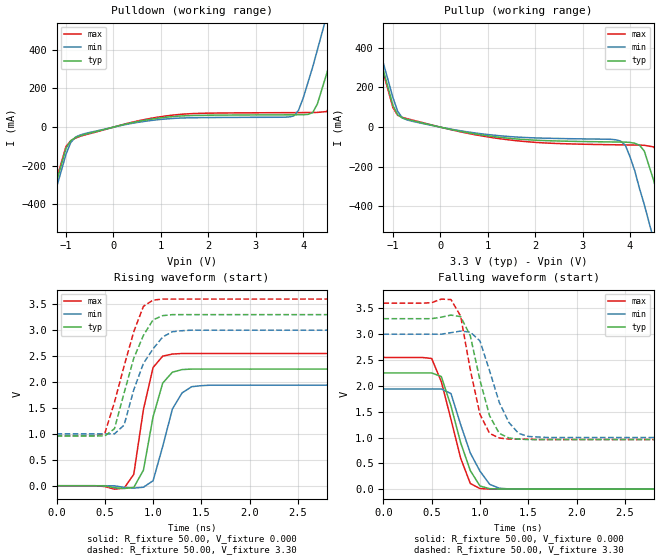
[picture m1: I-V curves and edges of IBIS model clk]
[IBIS Ver]   2.1
[File name]   66405.ibs
[File Rev]   1.0
[Date]   11/07/2011
[Source]   IDT CMD Applications Engineering
[Disclaimer] This information is for modeling purposes only, and is
(C) Copyright Integrated Circuit Systems, Inc. 1997-2004
   All rights reserved
ICS hereby grants the user of this IBIS model a non-exclusive,
nontransferable license to use this IBIS model under the following terms.
Before using this IBIS model, the user should read this license.
If the user does not accept these terms,  the IBIS model should be
returned to ICS within 30 days.
   The user is granted this license only to use the IBIS model and
is not granted rights to sell, load, rent, lease or license the IBIS
model in whole or in part, or in modified form to anyone other than
user. User may modify the IBIS model to suit its specific
applications but rights to derivative works and such modifications
shall belong to ICS.
   This IBIS model is provided on an "AS IS" basis and ICS makes
absolutely no warranty with respect to the information contained
herein. ICS DISCLAIMS AND CUSTOMER WAIVES ALL WARRANTIES, EXPRESS
OR IMPLIED, INCLUDING WARRANTIES OF MERCHANTABILITY OR FITNESS FOR
A PARTICULAR PURPOSE. The entire risk as to quality and performance
is with the Customer. ACCORDINGLY, IN NO EVENT SHALL THE COMPANY BE
LIABLE FOR ANY DAMAGES, WHETHER IN CONTRACT OR TORT,INCLUDING ANY
LOST PROFITS OR OTHER INCIDENTAL, CONSEQUENTIAL, EXEMPLARY, OR
PUNITIVE DAMAGES ARISING OUT OF THE USE OR APPLICATION OF THE IBIS
model provided in this package. Further, ICS reserves the right to
make changes without notice to any product herein to improve
reliability, function, or design. ICS does not convey any license
under patent rights or any other intellectual property rights,
including those of third parties.
   ICS is not obligated to provide maintenance or support
for the licensed IBIS model.
[Component]   ICS664-05
[Manufacturer] Integrated Circuit Systems Inc.
[Package]
|   typ   min   max
R_pkg   40m   35m   45m
L_pkg   1.65nH   1.35nH   1.95nH
C_pkg   0.24pF   0.14pF   0.34pF
[pin]   signal_name   model_name   R_pin   L_pin   C_pin
   9   CLK   clk
| Models and submodels in the file (1): clk (Output)
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|   ICS667 3.3V Clock Drive Model
| This model is suitable for all output pin on the
| ICS664-01
|   Model clk
[Model]   clk
Model_type   Output
Polarity   Non-Inverting
Vmeas =   1.65V
Cref =   5.00pF
Rref =  50.00
Vref =   1.65V
C_comp   5.50pF   5.00pF   6.00pF
[Temperature Range]   25.00   70.00   0.000
[Voltage Range]   3.30V   3.00V   3.60V
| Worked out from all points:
|   slope of the pulldown table from 0 to 0.495 V, typ, clamps not added: 17.6 ohm
|   slope of the pullup table from 0 to 0.495 V, typ, clamps not added: 20.3 ohm
|   rising waveform, R_fixture 50.00, V_fixture 0.000: 20-80 % time 158ps typ, 179ps min, 147ps max; typ from 0 V to 2.25 V
|   rising waveform, R_fixture 50.00, V_fixture 3.30: 20-80 % time 237ps typ, 252ps min, 241ps max; typ from 0.96 V to 3.3 V
|   falling waveform, R_fixture 50.00, V_fixture 0.000: 20-80 % time 217ps typ, 239ps min, 213ps max; typ from 2.25 V to 0 V
|   falling waveform, R_fixture 50.00, V_fixture 3.30: 20-80 % time 183ps typ, 225ps min, 169ps max; typ from 3.3 V to 0.96 V
[Pulldown]
| voltage   I(typ)   I(min)   I(max)
-3.3V     -2.25A     -2.28A     -2.24A
-1.5V     -540mA     -570mA     -520mA
-1V       -110mA     -140mA     -100mA
-700mV    -44.42mA   -40.49mA   -47.24mA
1.3V      55.66mA    45.68mA    63.49mA
3.8V      63.89mA    57.58mA    75.04mA
3.9V      64.06mA    85.93mA    75.17mA
4.2V      74.92mA    310mA      75.82mA
4.5V      280mA      580mA      80.87mA
4.7V      460mA      770mA      180mA
5.1V      830mA      1.14A      530mA
6.6V      2.26A      2.58A      1.96A
[Pullup]
| voltage   I(typ)   I(min)   I(max)
-3.3V     2.26A      2.29A      2.24A
-1.5V     550mA      580mA      530mA
-1V       110mA      150mA      99.39mA
-700mV    39.37mA    36.07mA    42.62mA
1.4V      -55.03mA   -46.42mA   -62.81mA
3.8V      -75.27mA   -70.05mA   -89.37mA
4V        -77.07mA   -150mA     -90.02mA
4.2V      -91.11mA   -310mA     -90.7mA
4.5V      -270mA     -570mA     -100mA
4.7V      -450mA     -760mA     -180mA
5.1V      -820mA     -1.14A     -520mA
6.6V      -2.26A     -2.57A     -1.95A
[Ramp]
| variable   typ   min   max
dV/dt_r   1.35/0.14n   1.16/0.16n   1.53/0.12n
dV/dt_f   1.40/0.18n   1.20/0.21n   1.58/0.16n
R_load = 50.00
[Rising Waveform]
R_fixture = 50.00
V_fixture = 0.000
V_fixture_min = 0.000
V_fixture_max = 0.000
| time   V(typ)   V(min)   V(max)
0s        0V         0V         0V
700ps     -53.64mV   -31.55mV   -47.01mV
800ps     -32.91mV   -45.92mV   220mV
900ps     300mV      -28.54mV   1.47V
1ns       1.33V      96.17mV    2.28V
1.1ns     1.98V      760mV      2.5V
1.2ns     2.19V      1.48V      2.54V
1.3ns     2.24V      1.79V      2.55V
1.4ns     2.25V      1.91V      2.55V
5ns       2.25V      1.94V      2.55V
[Rising Waveform]
R_fixture = 50.00
V_fixture = 3.30
V_fixture_min = 3.00
V_fixture_max = 3.60
| time   V(typ)   V(min)   V(max)
0s        960mV      1V         960mV
500ps     960mV      1V         1.01V
600ps     1.1V       1V         1.61V
700ps     1.79V      1.17V      2.31V
800ps     2.46V      1.85V      2.97V
900ps     2.9V       2.36V      3.46V
1ns       3.2V       2.64V      3.58V
1.2ns     3.3V       2.97V      3.6V
1.4ns     3.3V       3V         3.6V
5ns       3.3V       3V         3.6V
[Falling Waveform]
R_fixture = 50.00
V_fixture = 0.000
V_fixture_min = 0.000
V_fixture_max = 0.000
| time   V(typ)   V(min)   V(max)
0s        2.25V      1.94V      2.55V
500ps     2.25V      1.94V      2.53V
600ps     2.18V      1.94V      2.08V
700ps     1.61V      1.85V      1.35V
800ps     900mV      1.25V      600mV
900ps     360mV      700mV      110mV
1ns       61.1mV     350mV      11.47mV
1.1ns     9.52mV     94.71mV    2.23mV
1.3ns     1.1mV      4.55mV     810uV
5ns       3.1uV      8.72uV     1.49uV
[Falling Waveform]
R_fixture = 50.00
V_fixture = 3.30
V_fixture_min = 3.00
V_fixture_max = 3.60
| time   V(typ)   V(min)   V(max)
0s        3.3V       3V         3.6V
700ps     3.37V      3.03V      3.67V
800ps     3.34V      3.06V      3.35V
900ps     2.97V      3.04V      2.31V
1ns       2.11V      2.87V      1.45V
1.1ns     1.42V      2.29V      1.08V
1.2ns     1.08V      1.68V      990mV
1.3ns     990mV      1.29V      970mV
1.5ns     960mV      1.02V      970mV
5ns       960mV      1V         960mV
